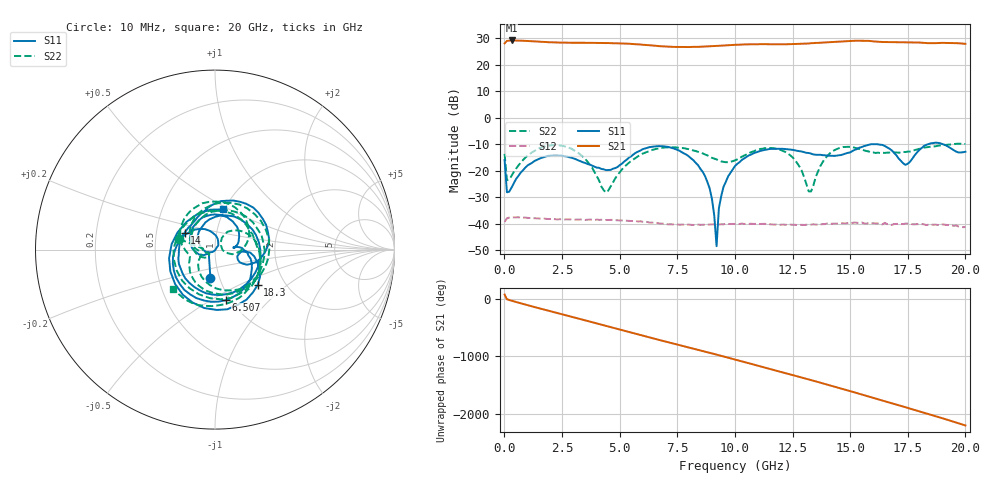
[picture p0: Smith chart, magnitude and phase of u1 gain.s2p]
!Keysight Technologies,P5004A,MY58100454,A.15.10.06
!Date: Monday, July 15, 2024 11:28:40
!Correction: S11(C  2-Port  )
!S21(C  2-Port  )
!S12(C  2-Port  )
!S22(C  2-Port  )
!S2P File: Measurements: S11, S21, S12, S22:
# Hz S  dB  R 50
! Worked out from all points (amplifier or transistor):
!   201 points, 10 MHz to 20 GHz, reference 50 ohm
!   highest |S21| = 29.2 dB at 309.9 MHz (marker M1)
!   |S21| within 3 dB of that: start of sweep to end of sweep
!   unconditionally stable (mu >= 1): start of sweep to end of sweep
!   at 3.308 GHz: K = 1.67, MAG = 28.6 dB, |S12| = -38.4 dB
!   at 10.01 GHz: K = 2.17, MAG = 27.7 dB, |S12| = -40.1 dB
!   at 20 GHz: K = 2.13, MAG = 28.5 dB, |S12| = -41.3 dB
!   S11 on the Smith chart (normalised r, x): 10 MHz: 0.91, -0.29; 6.507 GHz: 0.95, -0.59; 14 GHz: 0.70, +0.14; 18.3 GHz: 1.46, -0.63; 20 GHz: 0.99, +0.47
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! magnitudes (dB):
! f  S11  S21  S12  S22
! 10 MHz  -16.0  28.1  -39.3  -13.6
! 110 MHz  -28.1  29.0  -38.0  -23.6
! 309.9 MHz  -26.4  29.2  -37.6  -21.9
! 1.709 GHz  -14.9  28.6  -38.0  -10.9
! 3.408 GHz  -16.8  28.3  -38.4  -14.7
! 4.408 GHz  -19.8  28.2  -38.6  -28.2
! 6.507 GHz  -10.8  27.2  -39.7  -11.9
! 6.707 GHz  -10.7  27.0  -39.9  -11.6
! 8.606 GHz  -20.4  26.9  -40.4  -13.5
! 9.005 GHz  -30.7  27.0  -40.2  -15.1
! 9.205 GHz  -48.5  27.1  -40.2  -15.7
! 9.305 GHz  -34.2  27.2  -40.3  -16.1
! 9.405 GHz  -29.7  27.2  -40.2  -16.5
! 10.01 GHz  -18.2  27.5  -40.1  -16.1
! 12 GHz  -11.7  27.7  -40.4  -12.2
! 13.2 GHz  -13.3  28.0  -40.3  -27.8
! 13.4 GHz  -13.8  28.2  -40.2  -25.6
! 14 GHz  -14.3  28.5  -39.9  -14.5
! 16.7 GHz  -11.7  28.6  -40.1  -13.1
! 17.4 GHz  -17.8  28.5  -39.9  -12.9
! 18.3 GHz  -10.2  28.2  -40.5  -11.2
! 20 GHz  -12.8  27.9  -41.3  -9.9
